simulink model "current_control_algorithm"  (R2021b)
settings: Solver=FixedStepDiscrete  StartTime=0.0  StopTime=10.0  RelTol=1e-3
InitFcn:
  | foc_qep_data;
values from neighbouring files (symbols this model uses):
  PI_params = mcb.internal.SetControllerParameters(pmsm,inverter,PU_System,T_pwm,5*Ts,Ts_speed)    [foc_qep_data.m]
  pmsm = mcb_SetPMSMMotorParameters('BLY171D')    [foc_qep_data.m]
  PU_System = mcb_SetPUSystem(pmsm,inverter)    [foc_qep_data.m]
  Ts = T_pwm    (= 5e-05)    [foc_qep_data.m]    (also in open_loop_data.m; qep_calibration_data.m)
undefined symbols (not defined in the file or in its folder): bits, DiscIntNeverNeededParam, inverter, target
libraries: mcbcontrolslib x11, mcbpositiondecoderlib x3, simulink x2

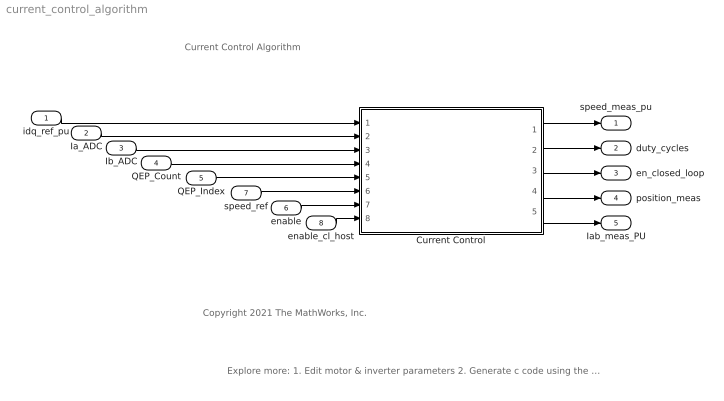
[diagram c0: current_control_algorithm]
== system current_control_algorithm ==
  note: Current Control Algorithm
  note: Explore more: 1. Edit motor & inverter parameters 2. Generate c code using the 'Embedded Coder' app 3. Integrate generated code with driver code 4. Control motor via host model
  note: Copyright 2021 The MathWorks, Inc.
  idq_ref_pu : Inport  OutDataTypeStr=dataType  PortDimensions=2
  Ia_ADC : Inport  Port=2  OutDataTypeStr=uint32
  Ib_ADC : Inport  Port=3  OutDataTypeStr=uint32
  QEP_Count : Inport  Port=4  OutDataTypeStr=uint16
  QEP_Index : Inport  Port=5  OutDataTypeStr=uint16
  enable : Inport  Port=6  OutDataTypeStr=boolean
  speed_ref : Inport  Port=7  OutDataTypeStr=dataType
  enable_cl_host : Inport  Port=8
  Current Control : Subsystem
  speed_meas_pu : Outport
  duty_cycles : Outport  Port=2
  en_closed_loop : Outport  Port=3
  position_meas : Outport  Port=4
  Iab_meas_PU : Outport  Port=5
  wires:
  idq_ref_pu/1 -> Current Control/1(Idq_ref_PU)
  Ia_ADC/1 -> Current Control/2(Ia_ADC)
  Ib_ADC/1 -> Current Control/3(Ib_ADC)
  QEP_Count/1 -> Current Control/4(QEP_Count)
  QEP_Index/1 -> Current Control/5(QEP_Index)
  enable/1 -> Current Control/7(enable)
  speed_ref/1 -> Current Control/6(speed_ref)
  Current Control/1(Speed_meas_PU) -> speed_meas_pu/1
  Current Control/2(Duty_Cycles) -> duty_cycles/1
  Current Control/3(en_closed_loop) -> en_closed_loop/1
  Current Control/4(position_meas) -> position_meas/1
  enable_cl_host/1 -> Current Control/8(enable_cl_host)
  Current Control/5(Iab_meas_PU) -> Iab_meas_PU/1

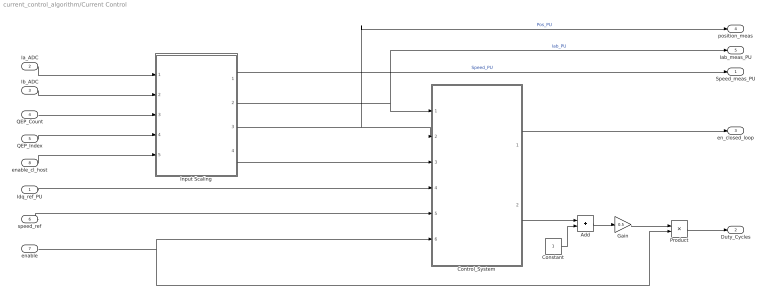
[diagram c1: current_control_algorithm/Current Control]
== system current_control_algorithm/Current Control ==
  Idq_ref_PU : Inport
  Ia_ADC : Inport  Port=2
  Ib_ADC : Inport  Port=3
  QEP_Count : Inport  Port=4
  QEP_Index : Inport  Port=5
  speed_ref : Inport  Port=6
  enable : Inport  Port=7
  enable_cl_host : Inport  Port=8
  Add : Sum
  Constant : Constant  OutDataTypeStr=dataType
  Control_System : Subsystem
  Gain : Gain  Gain=0.5
  Input Scaling : Subsystem
  Product : Product
  Speed_meas_PU : Outport  InitialOutput=0  VectorParamsAs1DForOutWhenUnconnected=off
  Duty_Cycles : Outport  Port=2
  en_closed_loop : Outport  Port=3
  position_meas : Outport  Port=4
  Iab_meas_PU : Outport  Port=5
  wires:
  Input Scaling/2(Iab_meas_PU) -> Iab_meas_PU/1, Control_System/1(Iab_meas_PU)  "Iab_PU"
  Input Scaling/3(Pos_PU) -> Control_System/2(Pos_PU), position_meas/1  "Pos_PU"
  Input Scaling/4(EnClosedLoop) -> Control_System/3(EnClosedLoop)
  Ia_ADC/1 -> Input Scaling/1(Ia_ADC)
  Ib_ADC/1 -> Input Scaling/2(Ib_ADC)
  QEP_Count/1 -> Input Scaling/3(QEP_Position_Count)
  QEP_Index/1 -> Input Scaling/4(QEP_Index_Latch)
  enable/1 -> Product/2, Control_System/6(enable)
  speed_ref/1 -> Control_System/5(speed_ref)
  Control_System/1(en_closed_loop) -> en_closed_loop/1
  Control_System/2(Duty_Cycles) -> Add/1
  Constant/1 -> Add/2
  Add/1 -> Gain/1
  Gain/1 -> Product/1
  Product/1 -> Duty_Cycles/1
  enable_cl_host/1 -> Input Scaling/5(enable_cl_host)
  Input Scaling/1(speed_PU) -> Speed_meas_PU/1  "Speed_PU"
  Idq_ref_PU/1 -> Control_System/4(Idq_ref_PU)

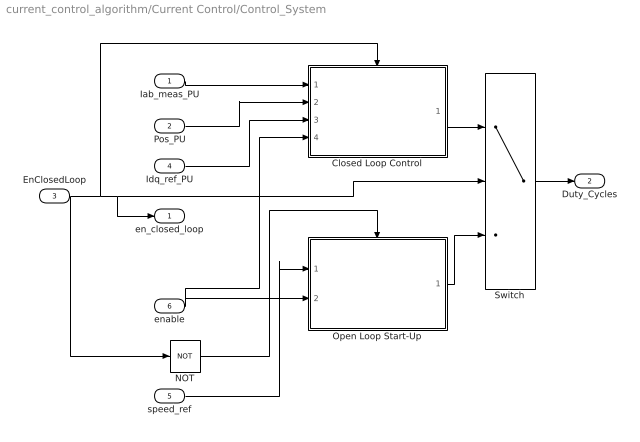
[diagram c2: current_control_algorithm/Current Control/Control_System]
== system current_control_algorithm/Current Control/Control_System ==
  Iab_meas_PU : Inport
  Pos_PU : Inport  Port=2
  EnClosedLoop : Inport  Port=3
  Idq_ref_PU : Inport  Port=4
  speed_ref : Inport  Port=5
  enable : Inport  Port=6
  Closed Loop Control : Subsystem
  NOT : Logic  Operator=NOT  IconShape=distinctive  AllPortsSameDT=off  OutDataTypeStr=boolean
  Open Loop Start-Up : Subsystem
  Switch : Switch  Criteria=u2 > Threshold  Threshold=0.5
  en_closed_loop : Outport
  Duty_Cycles : Outport  Port=2  VectorParamsAs1DForOutWhenUnconnected=off
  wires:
  speed_ref/1 -> Open Loop Start-Up/1(speed_ref)
  Open Loop Start-Up/1(PWM_Duty) -> Switch/3
  Pos_PU/1 -> Closed Loop Control/2(Pos_PU)
  Switch/1 -> Duty_Cycles/1
  NOT/1 -> Open Loop Start-Up/Enable
  Iab_meas_PU/1 -> Closed Loop Control/1(Iab_meas_PU)
  Idq_ref_PU/1 -> Closed Loop Control/3(Idq_ref_PU)
  Closed Loop Control/1(Vabc in PU) -> Switch/1
  enable/1 -> Closed Loop Control/4(enable), Open Loop Start-Up/2(enable)
  EnClosedLoop/1 -> Switch/2, en_closed_loop/1, Closed Loop Control/Enable, NOT/1

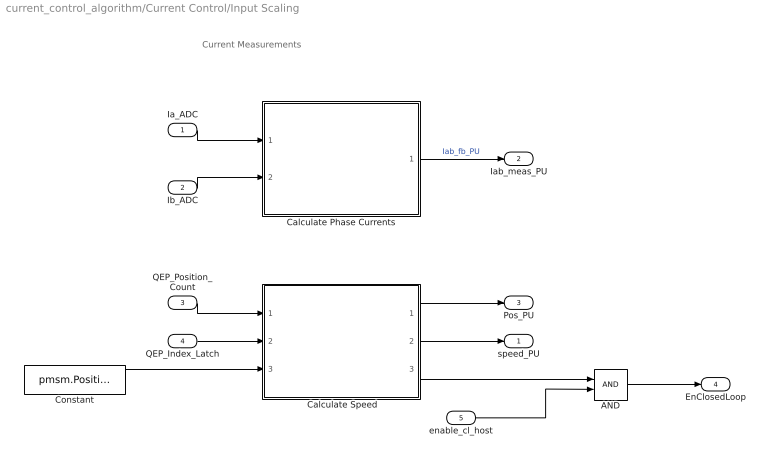
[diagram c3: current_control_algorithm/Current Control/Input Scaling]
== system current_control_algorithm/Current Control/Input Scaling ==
  note: Current Measurements
  Ia_ADC : Inport
  Ib_ADC : Inport  Port=2
  QEP_Position_Count : Inport  Port=3
  QEP_Index_Latch : Inport  Port=4
  enable_cl_host : Inport  Port=5
  " Calculate Speed" : Subsystem
  AND : Logic  IconShape=distinctive  AllPortsSameDT=off  OutDataTypeStr=boolean
  Calculate Phase Currents : Subsystem
  Constant : Constant  Value=pmsm.PositionOffset  OutDataTypeStr=dataType  SampleTime=-1
  speed_PU : Outport
  Iab_meas_PU : Outport  Port=2
  Pos_PU : Outport  Port=3
  EnClosedLoop : Outport  Port=4
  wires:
  " Calculate Speed"/2(speed) -> speed_PU/1
  Calculate Phase Currents/1(Iab_meas_PU) -> Iab_meas_PU/1  "Iab_fb_PU"
  QEP_Position_Count/1 -> " Calculate Speed"/1(QEP_Position_Count)
  " Calculate Speed"/1(Theta_e) -> Pos_PU/1
  Ia_ADC/1 -> Calculate Phase Currents/1(Ia_ADC)
  Ib_ADC/1 -> Calculate Phase Currents/2(Ib_ADC)
  Constant/1 -> " Calculate Speed"/3(Offset)
  QEP_Index_Latch/1 -> " Calculate Speed"/2(QEP_Index_Latch)
  " Calculate Speed"/3(IndexFound) -> AND/1
  enable_cl_host/1 -> AND/2
  AND/1 -> EnClosedLoop/1

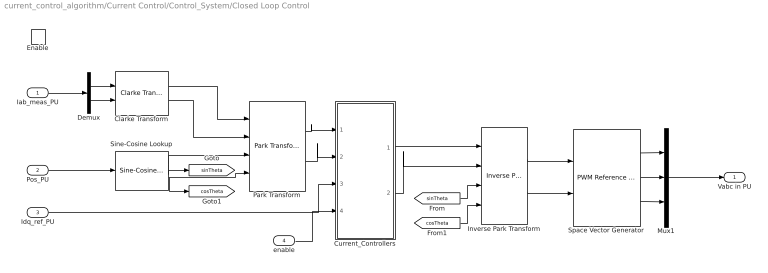
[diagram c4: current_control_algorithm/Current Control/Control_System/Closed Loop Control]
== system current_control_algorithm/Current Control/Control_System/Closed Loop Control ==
  Iab_meas_PU : Inport
  Pos_PU : Inport  Port=2
  Idq_ref_PU : Inport  Port=3
  enable : Inport  Port=4
  Enable : EnablePort
  Clarke Transform : mcbcontrolslib/Clarke Transform  VariantControl=Variant2
  Current_Controllers : Subsystem
  Demux : Demux  Outputs=2
  Inverse Park Transform : mcbcontrolslib/Inverse Park Transform  AxisAlignment=D-axis
  Mux1 : Mux  Inputs=3
  Park Transform : mcbcontrolslib/Park Transform  AxisAlignment=D-axis
  Sine-Cosine Lookup : mcbcontrolslib/Sine-Cosine Lookup  AngleInput=Per-unit  N_points=1024
  Space Vector Generator : mcbcontrolslib/PWM Reference Generator  inSignal=Valphabeta  modType=SVM: space vector modulation
  Vabc in PU : Outport  VectorParamsAs1DForOutWhenUnconnected=off
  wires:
  Current_Controllers/1(Vd_ref) -> Inverse Park Transform/1
  Inverse Park Transform/1 -> Space Vector Generator/1
  Park Transform/1 -> Current_Controllers/1(Id)
  Clarke Transform/1 -> Park Transform/1
  [sinTheta] -> Inverse Park Transform/3
  Sine-Cosine Lookup/1 -> [sinTheta], Park Transform/3
  Clarke Transform/2 -> Park Transform/2
  Space Vector Generator/1 -> Mux1/1
  Space Vector Generator/3 -> Mux1/3
  Sine-Cosine Lookup/2 -> Park Transform/4, [cosTheta]
  Space Vector Generator/2 -> Mux1/2
  Idq_ref_PU/1 -> Current_Controllers/3(Idq_ref_PU)
  Iab_meas_PU/1 -> Demux/1
  Inverse Park Transform/2 -> Space Vector Generator/2
  Demux/1 -> Clarke Transform/1
  Demux/2 -> Clarke Transform/2
  Park Transform/2 -> Current_Controllers/2(Iq)
  [cosTheta] -> Inverse Park Transform/4
  Pos_PU/1 -> Sine-Cosine Lookup/1
  Current_Controllers/2(Vq_ref) -> Inverse Park Transform/2
  Mux1/1 -> Vabc in PU/1
  enable/1 -> Current_Controllers/4(enable)

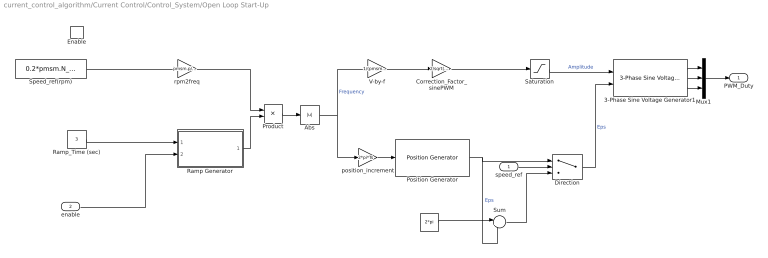
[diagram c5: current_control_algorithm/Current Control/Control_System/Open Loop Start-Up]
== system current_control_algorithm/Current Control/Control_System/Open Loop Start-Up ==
  speed_ref : Inport
  enable : Inport  Port=2
  Enable : EnablePort
  " " : Constant  Value=2*pi  OutDataTypeStr=dataType  SampleTime=-1
  3-Phase Sine Voltage Generator1 : mcbcontrolslib/3-Phase Sine Voltage Generator  AngleInput=Radians  N_points=1024
  Abs : Abs
  Correction_Factor_sinePWM : Gain  Gain=2/sqrt(3)  RndMeth=Simplest
  Direction : Switch  Criteria=u2 > Threshold  OutDataTypeStr=dataType  RndMeth=Simplest
  Mux1 : Mux  Inputs=3
  Position Generator : mcbcontrolslib/Position Generator  AngleOutput=Radians  ThetaSource=External  ThetaInput=5e-4  DataType=double  ExternalReset=none
  Product : Product  RndMeth=Simplest
  Ramp Generator : Subsystem
  Ramp_Time (sec) : Constant  Value=3  OutDataTypeStr=dataType  SampleTime=-1
  Saturation : Saturate  UpperLimit=0.95  LowerLimit=0.15  RndMeth=Simplest
  Speed_ref(rpm) : Constant  Value=0.2*pmsm.N_base  OutDataTypeStr=dataType  SampleTime=-1
  Sum : Sum  Inputs=|+-  RndMeth=Simplest
  V-by-f : Gain  Gain=1/(pmsm.N_base*pmsm.p*2/120)  RndMeth=Simplest
  position_increment : Gain  Gain=2*pi*Ts  RndMeth=Simplest
  rpm2freq : Gain  Gain=pmsm.p/60  RndMeth=Simplest
  PWM_Duty : Outport  VectorParamsAs1DForOutWhenUnconnected=off
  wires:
  3-Phase Sine Voltage Generator1/1 -> Mux1/1
  3-Phase Sine Voltage Generator1/3 -> Mux1/3
  Direction/1 -> 3-Phase Sine Voltage Generator1/2  "Eps"
  Speed_ref(rpm)/1 -> rpm2freq/1
  Saturation/1 -> 3-Phase Sine Voltage Generator1/1  "Amplitude"
  Mux1/1 -> PWM_Duty/1
  Ramp Generator/1(Ramp) -> Product/2
  Ramp_Time (sec)/1 -> Ramp Generator/1(Ramp_Time)
  Position Generator/1 -> Direction/1, Sum/2  "Eps"
  " "/1 -> Sum/1
  Sum/1 -> Direction/3
  Abs/1 -> position_increment/1, V-by-f/1  "Frequency"
  position_increment/1 -> Position Generator/1
  V-by-f/1 -> Correction_Factor_sinePWM/1
  Product/1 -> Abs/1
  rpm2freq/1 -> Product/1
  speed_ref/1 -> Direction/2
  Correction_Factor_sinePWM/1 -> Saturation/1
  3-Phase Sine Voltage Generator1/2 -> Mux1/2
  enable/1 -> Ramp Generator/2(Enable)

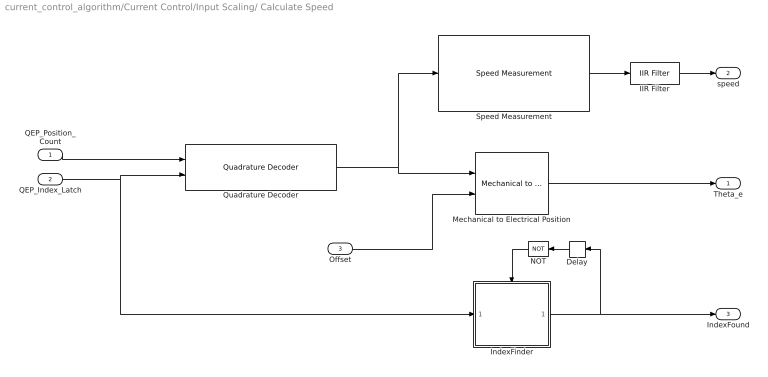
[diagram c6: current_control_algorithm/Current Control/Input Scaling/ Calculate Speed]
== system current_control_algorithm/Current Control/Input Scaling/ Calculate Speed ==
  QEP_Position_Count : Inport
  QEP_Index_Latch : Inport  Port=2
  Offset : Inport  Port=3
  Delay : Delay  DelayLength=1
  IIR Filter : mcbcontrolslib/IIR Filter  VariantControl=Low Pass Filter  VariantSelect=Low-pass  Filter_constant=0.01  advancedSettings=off  Ts=50e-6  cutOff_freq=32.1525
  IndexFinder : Subsystem
  Mechanical to Electrical Position : mcbpositiondecoderlib/Mechanical to Electrical Position  NrPP=pmsm.p  selectedRange=Per unit  MechOfstInputType=Input port  mechOffsetIn=0  maxAngleIn=1  InputDataType=dataType  VariantSelect=floating-point
  NOT : Logic  Operator=NOT  AllPortsSameDT=off  OutDataTypeStr=boolean
  Quadrature Decoder : mcbpositiondecoderlib/Quadrature Decoder  EncoderSlitsPerRevolution=pmsm.QEPSlits  EncoderCountsPerSlit=4  CounterSize=16 bits  ExternalIndexCount=on  PositionUnit=Per unit  PositionDataType=dataType
  Speed Measurement : mcbpositiondecoderlib/Speed Measurement  PositionUnit=Per unit  PositionScalingDatatype=uint32  SpeedCalculationMode=Time interval for speed calculation  SampleTimeAsync=Ts  MaximumApplicationSpeed=6000  SpeedResolution=5e-6  DelayLength=20  MaximumMeasurableSpeed=29999  MeasurableSpeedResolution=1.397e-05  SpeedUnit=Per unit based on dialog  PerUnitSpeed=PU_System.N_base  SpeedDataType=dataType
  Theta_e : Outport  VectorParamsAs1DForOutWhenUnconnected=off
  speed : Outport  Port=2  VectorParamsAs1DForOutWhenUnconnected=off
  IndexFound : Outport  Port=3  InitialOutput=0  VectorParamsAs1DForOutWhenUnconnected=off
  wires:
  Mechanical to Electrical Position/1 -> Theta_e/1
  Speed Measurement/1 -> IIR Filter/1
  Quadrature Decoder/1 -> Speed Measurement/1, Mechanical to Electrical Position/1
  QEP_Position_Count/1 -> Quadrature Decoder/1
  Offset/1 -> Mechanical to Electrical Position/2
  IIR Filter/1 -> speed/1
  NOT/1 -> IndexFinder/Enable
  IndexFinder/1(Out1) -> Delay/1, IndexFound/1
  QEP_Index_Latch/1 -> IndexFinder/1(In1), Quadrature Decoder/2
  Delay/1 -> NOT/1

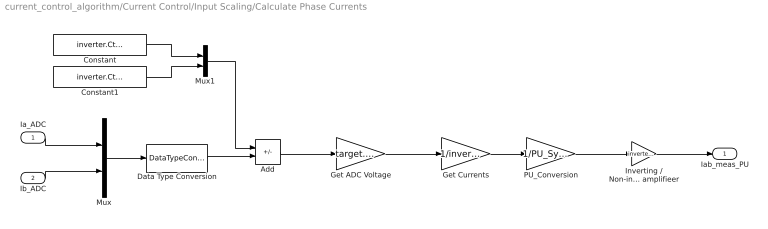
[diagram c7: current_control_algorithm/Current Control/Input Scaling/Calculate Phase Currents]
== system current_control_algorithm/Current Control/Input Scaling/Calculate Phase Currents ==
  Ia_ADC : Inport
  Ib_ADC : Inport  Port=2
  Add : Sum  Inputs=-+
  Constant : Constant  Value=inverter.CtSensAOffset  OutDataTypeStr=Inherit: Inherit via back propagation
  Constant1 : Constant  Value=inverter.CtSensBOffset  OutDataTypeStr=Inherit: Inherit via back propagation
  Data Type Conversion : DataTypeConversion  OutDataTypeStr=int32  ConvertRealWorld=Stored Integer (SI)
  Get ADC Voltage : Gain  Gain=target.ADC_Vref /target.ADC_MaxCount  OutDataTypeStr=dataType  RndMeth=Simplest
  Get Currents : Gain  Gain=1/inverter.ISenseVoltPerAmp  RndMeth=Simplest
  Inverting / Non-inverting Current measurement amplifieer : Gain  Gain=inverter.invertingAmp  RndMeth=Simplest
  Mux : Mux  Inputs=2
  Mux1 : Mux  Inputs=2
  PU_Conversion : Gain  Gain=1/PU_System.I_base  RndMeth=Simplest
  Iab_meas_PU : Outport  VectorParamsAs1DForOutWhenUnconnected=off
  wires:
  Mux1/1 -> Add/1
  Data Type Conversion/1 -> Add/2
  Ia_ADC/1 -> Mux/1
  Ib_ADC/1 -> Mux/2
  Mux/1 -> Data Type Conversion/1
  PU_Conversion/1 -> Inverting / Non-inverting Current measurement amplifieer/1
  Constant/1 -> Mux1/1
  Constant1/1 -> Mux1/2
  Inverting / Non-inverting Current measurement amplifieer/1 -> Iab_meas_PU/1
  Get ADC Voltage/1 -> Get Currents/1
  Add/1 -> Get ADC Voltage/1
  Get Currents/1 -> PU_Conversion/1

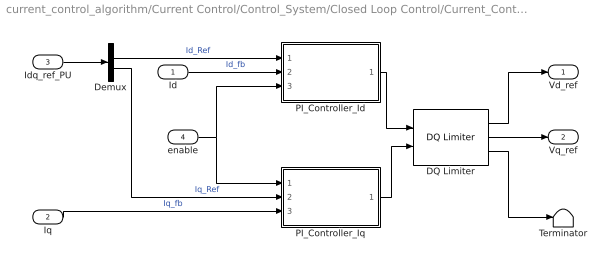
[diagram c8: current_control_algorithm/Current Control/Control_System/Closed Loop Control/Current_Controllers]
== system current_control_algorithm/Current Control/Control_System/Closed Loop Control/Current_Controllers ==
  Id : Inport
  Iq : Inport  Port=2
  Idq_ref_PU : Inport  Port=3
  enable : Inport  Port=4
  DQ Limiter : mcbcontrolslib/DQ Limiter  Vmax=0.95
  Demux : Demux  Outputs=2
  PI_Controller_Id : Subsystem
  PI_Controller_Iq : Subsystem
  Terminator : Terminator
  Vd_ref : Outport  VectorParamsAs1DForOutWhenUnconnected=off
  Vq_ref : Outport  Port=2  VectorParamsAs1DForOutWhenUnconnected=off
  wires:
  Iq/1 -> PI_Controller_Iq/3(I_fb)  "Iq_fb"
  Id/1 -> PI_Controller_Id/2(I_fb)  "Id_fb"
  Demux/1 -> PI_Controller_Id/1(I_ref)  "Id_Ref"
  Demux/2 -> PI_Controller_Iq/2(I_ref)  "Iq_Ref"
  Idq_ref_PU/1 -> Demux/1
  PI_Controller_Id/1(V_ref) -> DQ Limiter/1
  PI_Controller_Iq/1(V_ref) -> DQ Limiter/2
  DQ Limiter/1 -> Vd_ref/1
  DQ Limiter/2 -> Vq_ref/1
  DQ Limiter/3 -> Terminator/1
  enable/1 -> PI_Controller_Iq/1(enable), PI_Controller_Id/3(enable)

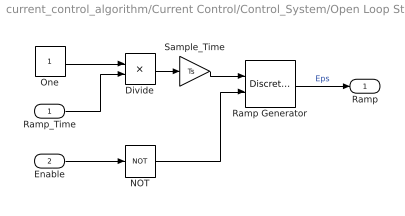
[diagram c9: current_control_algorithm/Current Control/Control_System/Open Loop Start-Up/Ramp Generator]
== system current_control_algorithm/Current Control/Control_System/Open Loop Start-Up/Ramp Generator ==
  Ramp_Time : Inport
  Enable : Inport  Port=2
  Divide : Product  Inputs=*/  RndMeth=Simplest
  NOT : Logic  Operator=NOT  IconShape=distinctive  AllPortsSameDT=off  OutDataTypeStr=boolean
  One : Constant  OutDataTypeStr=single  SampleTime=-1
  Ramp Generator : DiscreteIntegrator  IntegratorMethod=Accumulation: Forward Euler  gainval=1  ExternalReset=sampled level  SampleTime=-1  OutDataTypeStr=single  RndMeth=Simplest  LimitOutput=on  UpperSaturationLimit=1  LowerSaturationLimit=0  ICPrevOutput=DiscIntNeverNeededParam  ICPrevScaledInput=DiscIntNeverNeededParam
  Sample_Time : Gain  Gain=Ts  RndMeth=Simplest
  Ramp : Outport
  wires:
  Divide/1 -> Sample_Time/1
  Ramp Generator/1 -> Ramp/1  "Eps"
  Sample_Time/1 -> Ramp Generator/1
  One/1 -> Divide/1
  Ramp_Time/1 -> Divide/2
  Enable/1 -> NOT/1
  NOT/1 -> Ramp Generator/2

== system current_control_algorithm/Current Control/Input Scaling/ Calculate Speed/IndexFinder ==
  In1 : Inport
  Enable : EnablePort
  AND : Logic  Inputs=3  AllPortsSameDT=off  OutDataTypeStr=boolean
  Compare To Constant : simulink/Logic and Bit Operations/Compare To Constant  relop===  const=0  OutDataTypeStr=boolean
  Compare To Constant1 : simulink/Logic and Bit Operations/Compare To Constant  relop=>  const=0  OutDataTypeStr=boolean
  Constant : Constant  OutDataTypeStr=boolean
  Delay3 : Delay  DelayLength=1
  Out1 : Outport
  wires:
  In1/1 -> Delay3/1, Compare To Constant1/1
  Compare To Constant1/1 -> AND/2
  Compare To Constant/1 -> AND/1
  Delay3/1 -> Compare To Constant/1
  AND/1 -> Out1/1
  Constant/1 -> AND/3

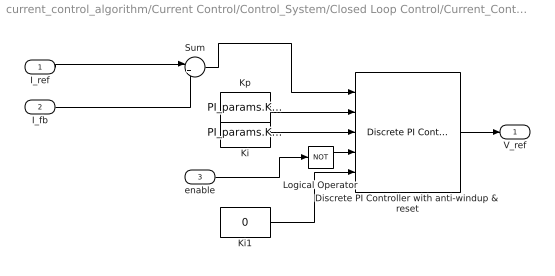
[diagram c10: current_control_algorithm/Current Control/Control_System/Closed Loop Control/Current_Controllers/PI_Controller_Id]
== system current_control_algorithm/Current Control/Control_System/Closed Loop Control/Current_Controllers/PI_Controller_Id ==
  I_ref : Inport
  I_fb : Inport  Port=2
  enable : Inport  Port=3
  Discrete PI Controller with anti-windup & reset : mcbcontrolslib/Discrete PI Controller  with anti-windup & reset  UpperSaturationLimit=1  LowerSaturationLimit=-1
  Ki : Constant  Value=PI_params.Ki_i*Ts  OutDataTypeStr=dataType  SampleTime=-1
  Ki1 : Constant  Value=0  OutDataTypeStr=dataType  SampleTime=-1
  Kp : Constant  Value=PI_params.Kp_i  OutDataTypeStr=dataType  SampleTime=-1
  Logical Operator : Logic  Operator=NOT  IconShape=distinctive  AllPortsSameDT=off  OutDataTypeStr=boolean
  Sum : Sum  Inputs=|+-
  V_ref : Outport  VectorParamsAs1DForOutWhenUnconnected=off
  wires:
  I_ref/1 -> Sum/1
  I_fb/1 -> Sum/2
  enable/1 -> Logical Operator/1
  Discrete PI Controller with anti-windup & reset/1 -> V_ref/1
  Sum/1 -> Discrete PI Controller with anti-windup & reset/1
  Kp/1 -> Discrete PI Controller with anti-windup & reset/2
  Ki/1 -> Discrete PI Controller with anti-windup & reset/3
  Logical Operator/1 -> Discrete PI Controller with anti-windup & reset/4
  Ki1/1 -> Discrete PI Controller with anti-windup & reset/5

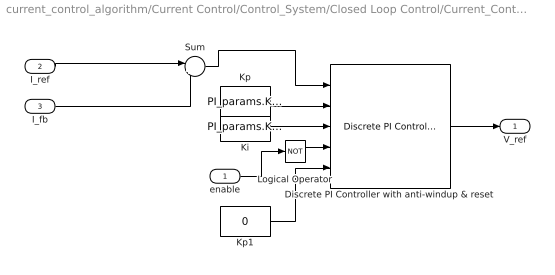
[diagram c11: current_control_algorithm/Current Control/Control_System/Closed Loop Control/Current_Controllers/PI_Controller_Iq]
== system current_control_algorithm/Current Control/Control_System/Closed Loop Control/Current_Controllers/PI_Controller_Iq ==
  enable : Inport
  I_ref : Inport  Port=2
  I_fb : Inport  Port=3
  Discrete PI Controller with anti-windup & reset : mcbcontrolslib/Discrete PI Controller  with anti-windup & reset  UpperSaturationLimit=1  LowerSaturationLimit=-1
  Ki : Constant  Value=PI_params.Ki_i*Ts  OutDataTypeStr=dataType  SampleTime=-1
  Kp : Constant  Value=PI_params.Kp_i  OutDataTypeStr=dataType  SampleTime=-1
  Kp1 : Constant  Value=0  OutDataTypeStr=dataType  SampleTime=-1
  Logical Operator : Logic  Operator=NOT  IconShape=distinctive  AllPortsSameDT=off  OutDataTypeStr=boolean
  Sum : Sum  Inputs=|+-
  V_ref : Outport  VectorParamsAs1DForOutWhenUnconnected=off
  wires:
  Discrete PI Controller with anti-windup & reset/1 -> V_ref/1
  enable/1 -> Logical Operator/1
  I_fb/1 -> Sum/2
  I_ref/1 -> Sum/1
  Kp/1 -> Discrete PI Controller with anti-windup & reset/2
  Sum/1 -> Discrete PI Controller with anti-windup & reset/1
  Ki/1 -> Discrete PI Controller with anti-windup & reset/3
  Logical Operator/1 -> Discrete PI Controller with anti-windup & reset/4
  Kp1/1 -> Discrete PI Controller with anti-windup & reset/5
